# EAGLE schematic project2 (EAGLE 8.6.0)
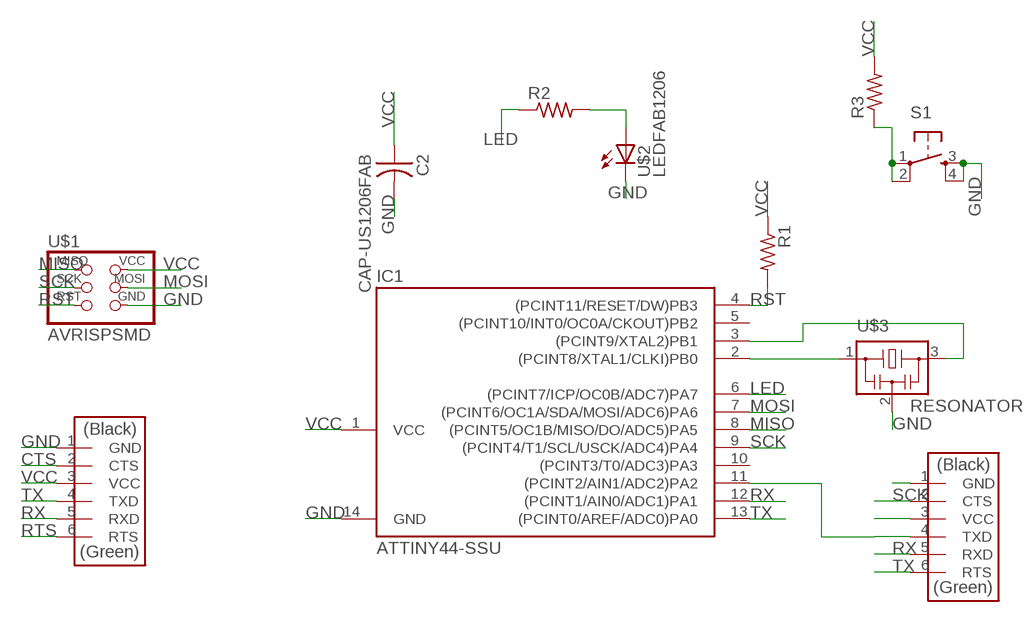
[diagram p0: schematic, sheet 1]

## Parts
C2  CAP-US1206FAB  [C1206FAB]
IC1  ATTINY44-SSU  [SOIC14]
R1  RES-US1206FAB  [R1206FAB]
R2  RES-US1206FAB  [R1206FAB]
R3  RES-US1206FAB  [R1206FAB]
S1  6MM_SWITCH6MM_SWITCH  [6MM_SWITCH]
U$1  AVRISPSMD  [2X03SMD]
U$2  LEDFAB1206  [LED1206FAB]
U$3  RESONATOR  [EFOBM]
U$4  FTDI-SMD-HEADER  [1X06SMD]
U$5  FTDI-SMD-HEADER  [1X06SMD]

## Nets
CTS: U$4.2(CTS)
GND: C2.2 IC1.14(GND) S1.3(S) S1.4(S1) U$1.6(GND) U$2.2(C) U$3.2 U$4.1(GND) U$5.1(GND)
LED: IC1.6((PCINT7/ICP/OC0B/ADC7)PA7) R2.1
MISO: IC1.8((PCINT5/OC1B/MISO/DO/ADC5)PA5) U$1.1(MISO)
MOSI: IC1.7((PCINT6/OC1A/SDA/MOSI/ADC6)PA6) U$1.4(MOSI)
N$1: R2.2 U$2.1(A)
N$2: R3.1 S1.1(P) S1.2(P1)
N$3: IC1.3((PCINT9/XTAL2)PB1) U$3.3
N$4: IC1.2((PCINT8/XTAL1/CLKI)PB0) U$3.1
N$8: IC1.11((PCINT2/AIN1/ADC2)PA2) U$5.4(TXD)
RST: IC1.4((PCINT11/RESET/DW)PB3) R1.2 U$1.5(RST)
RTS: U$4.6(RTS)
RX: IC1.12((PCINT1/AIN0/ADC1)PA1) U$4.5(RXD) U$5.5(RXD)
SCK: IC1.9((PCINT4/T1/SCL/USCK/ADC4)PA4) U$1.3(SCK) U$5.2(CTS)
TX: IC1.13((PCINT0/AREF/ADC0)PA0) U$4.4(TXD) U$5.6(RTS)
VCC: C2.1 IC1.1(VCC) R1.1 R3.2 U$1.2(VCC) U$4.3(VCC) U$5.3(VCC)
Unconnected: IC1.5((PCINT10/INT0/OC0A/CKOUT)PB2) IC1.10((PCINT3/T0/ADC3)PA3)

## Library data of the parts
C2 = fab:CAP-US
IC1 = fab:ATTINY44
R1-R3 = fab:RES-US: Resistor (US Symbol)
S1 = fab:6MM_SWITCH: OMRON SWITCH
U$1 = fab:AVRISP
U$2 = fab:LED: LED
U$3 = fab:RESONATOR
U$4 U$5 = fab:FTDI-SMD-HEADER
